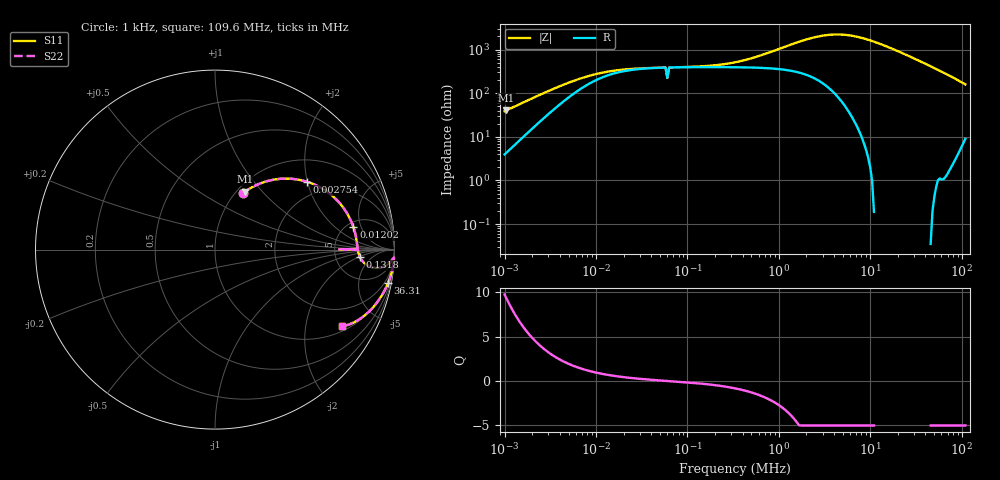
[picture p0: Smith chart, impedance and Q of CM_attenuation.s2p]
! EM Consulting and Software
! Touchstone file was created on 2026-03-05  19:00:36
# HZ S RI R 50.0000
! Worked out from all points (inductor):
!   253 points, 1 kHz to 109.6 MHz, reference 50 ohm
!   read as one part in series: L = 6.08 mH near 1.047 kHz
!   highest Q = 9.29 at 1.047 kHz (marker M1), where L = 6.12 mH
!   self-resonance near 61.28 kHz
!   S11 on the Smith chart (normalised r, x): 1 kHz: 1.08, +0.77; 2.754 kHz: 1.56, +1.99; 12.02 kHz: 5.72, +3.68; 131.8 kHz: 8.92, -2.09; 36.31 MHz: 1, -10; 109.6 MHz: 1.18, -3.18
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1000  0.1541 0.3133  0.8459 -0.3133  0.8459 -0.3133  0.1541 0.3133
1047.129  0.1658 0.322  0.8342 -0.322  0.8342 -0.322  0.1658 0.322
1737.801  0.3341 0.3908  0.6659 -0.3908  0.6659 -0.3908  0.3341 0.3908
2754.229  0.5126 0.3779  0.4874 -0.3779  0.4874 -0.3779  0.5126 0.3779
4365.158  0.6512 0.302  0.3488 -0.302  0.3488 -0.302  0.6512 0.302
6918.31  0.7298 0.2119  0.2702 -0.2119  0.2702 -0.2119  0.7298 0.2119
12022.64  0.771 0.1254  0.229 -0.1254  0.229 -0.1254  0.771 0.1254
47863.01  0.7936 0.0133  0.2064 -0.0133  0.2064 -0.0133  0.7936 0.0133
57543.99  0.7949 0.00363  0.2051 -0.00363  0.2051 -0.00363  0.7949 0.00363
60255.96  0.6916 0.00144  0.3084 -0.00144  0.3084 -0.00144  0.6916 0.00144
63095.73  0.7957 -0.00112  0.2043 0.00112  0.2043 0.00112  0.7957 -0.00112
131825.7  0.8071 -0.0407  0.1929 0.0407  0.1929 0.0407  0.8071 -0.0407
331131.1  0.8588 -0.0929  0.1412 0.0929  0.1412 0.0929  0.8588 -0.0929
630957.3  0.9229 -0.1003  0.0771 0.1003  0.0771 0.1003  0.9229 -0.1003
2290868  0.9904 -0.0528  0.00964 0.0528  0.00964 0.0528  0.9904 -0.0528
3630781  0.9954 -0.0453  0.00465 0.0453  0.00465 0.0453  0.9954 -0.0453
5754399  0.997 -0.0466  0.00303 0.0466  0.00303 0.0466  0.997 -0.0466
9120108  0.9965 -0.0577  0.0035 0.0577  0.0035 0.0577  0.9965 -0.0577
1.659587e7  0.9918 -0.0911  0.0082 0.0911  0.0082 0.0911  0.9918 -0.0911
3.630781e7  0.9647 -0.185  0.0353 0.185  0.0353 0.185  0.9647 -0.185
6.91831e7  0.878 -0.3247  0.122 0.3247  0.122 0.3247  0.878 -0.3247
1.096478e8  0.7063 -0.4279  0.2937 0.4279  0.2937 0.4279  0.7063 -0.4279
